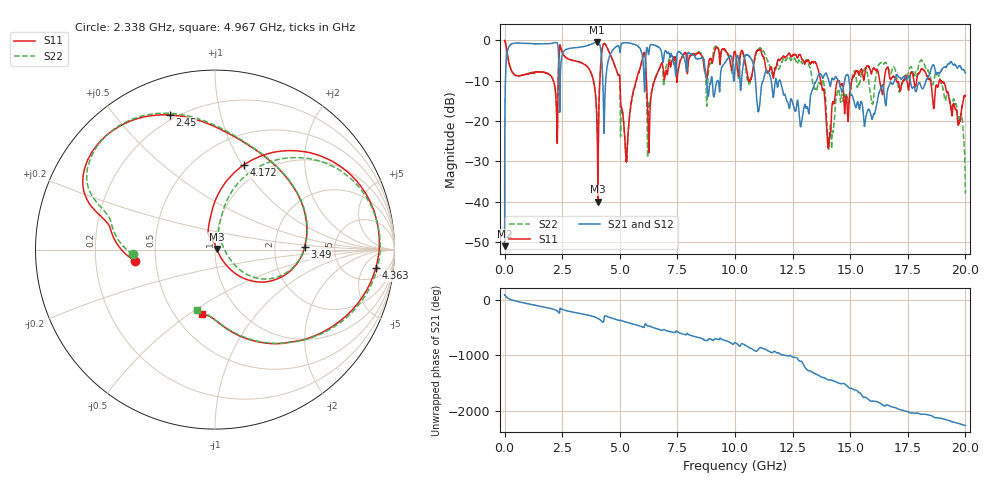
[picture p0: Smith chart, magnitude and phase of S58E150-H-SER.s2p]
!{S58E150}
!Johanson Technology Inc.
!www.johansontechnology.com
!Test Board Conditions:
!Substrate Type  RO4350B
!Substrate Thickness  60 mil
!Substrate Dk  3.66
!TL Type: GCPW
!TL Trace Width  115 mil
!TL Gap  52 mil
!Electrode orientation  Horizontal
!DUT TOPOLOGY	SERIES
!Mounting Pad LxW  55x428 mil
! Created Wed Apr 14 11:12:42 2021
# mhz S ma R 50
! 2 Port Network Data from SP1.SP block
! freq  magS11  angS11  magS21  angS21  magS12  angS12  magS22  angS22
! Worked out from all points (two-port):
!   20001 points, 300 kHz to 20 GHz, reference 50 ohm
!   highest |S21| = -0.37 dB at 4.021 GHz (marker M1); lowest = -51.0 dB at 300 kHz (marker M2)
!   |S21| within 3 dB of the highest: 103 MHz to 2.338 GHz (2.235 GHz wide, 183 % of centre); 2.507 GHz to 4.196 GHz (1.688 GHz wide, 50.4 % of centre)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
!   lowest |S11| = -40.0 dB at 4.049 GHz (marker M3), VSWR 1.02, Z = 50.9 + j0.383 ohm
!   |S11| at or under -10 dB: 5.006 GHz to 5.71 GHz (704.2 MHz wide, 13.1 % of centre); 13.72 GHz to 14.46 GHz (739.4 MHz wide, 5.25 % of centre); 18.93 GHz to end of sweep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
!   |S22| runs from -38.0 to 0.0 dB; largest |S21 - S12| = 0.0094
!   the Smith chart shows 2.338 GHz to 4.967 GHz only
!   S11 on the Smith chart (normalised r, x): 2.338 GHz: 0.38, -0.06; 2.45 GHz: 0.18, +0.71; 3.49 GHz: 2.99, +0.13; 4.172 GHz: 0.81, +1.02; 4.363 GHz: 9, -10; 4.967 GHz: 0.68, -0.57
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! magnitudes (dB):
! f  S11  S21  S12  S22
! 300 kHz  0.0  -51.0  -51.0  0.0
! 212.3 MHz  -6.0  -1.3  -1.3  -6.0
! 2.338 GHz  -6.9  -3.4  -3.4  -6.8
! 2.45 GHz  -2.0  -5.3  -5.2  -2.1
! 3.334 GHz  -5.5  -1.6  -1.6  -5.5
! 3.49 GHz  -6.0  -1.5  -1.5  -6.0
! 4.021 GHz  -23.2  -0.4  -0.4  -21.7
! 4.049 GHz  -40.0  -0.4  -0.4  -26.3
! 4.172 GHz  -6.1  -2.2  -2.2  -5.9
! 4.363 GHz  -0.9  -12.7  -12.7  -0.9
! 4.967 GHz  -8.7  -1.5  -1.5  -9.1
! 5.284 GHz  -30.1  -0.6  -0.6  -29.9
! 5.996 GHz  -4.2  -4.4  -4.4  -4.1
! 6.273 GHz  -25.8  -2.9  -2.9  -16.2
! 6.667 GHz  -7.6  -1.6  -1.6  -7.7
! 10 GHz  -2.8  -7.1  -7.1  -3.0
! 13.33 GHz  -5.3  -12.6  -12.6  -9.1
! 14.07 GHz  -25.9  -9.9  -9.9  -26.9
! 14.46 GHz  -10.0  -9.9  -9.8  -12.3
! 16.67 GHz  -7.5  -11.5  -11.5  -7.0
! 18.8 GHz  -11.5  -8.0  -8.0  -8.5
! 20 GHz  -13.8  -8.1  -8.0  -38.0
